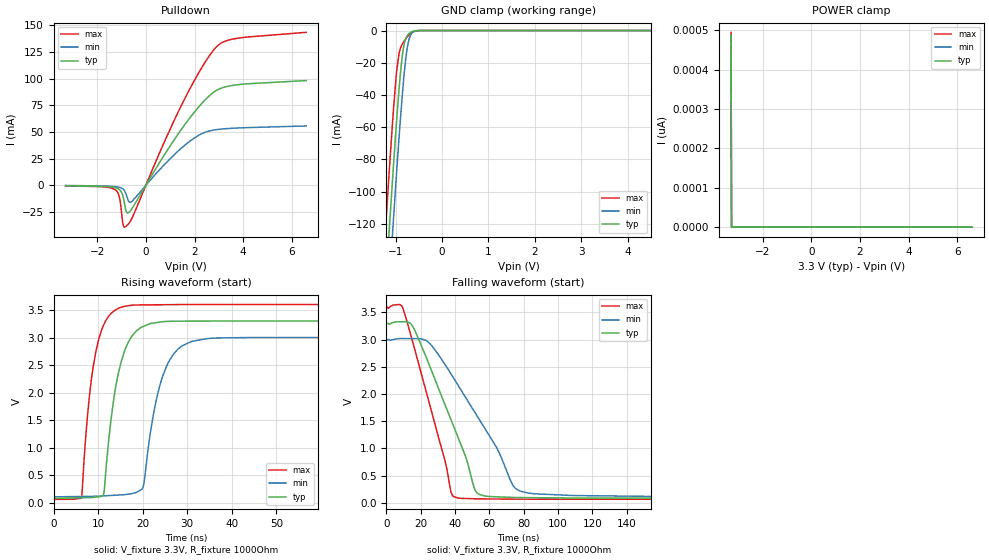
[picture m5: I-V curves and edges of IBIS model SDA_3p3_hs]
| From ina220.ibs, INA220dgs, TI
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|   Model
[Model]   SDA_3p3_hs
Model_type   I/O_open_drain
Polarity   Non-Inverting
Enable   Active-Low
Vinl = 0.99
Vinh = 2.31
Vmeas = 1.65
Vref = 3.3
Cref = 1pF
Rref = 1000
|   typ   min   max
C_comp   2.2433820E-12   1.9359850E-12 2.5433970E-12
[Voltage Range]   3.3   3   3.6
[Temperature Range]   27   85   -40
[Pullup Reference]   3.3   3   3.6
[Pulldown Reference]   -0   -0   -0
[Power Clamp Reference]   3.3   3   3.6
[GND Clamp Reference]   -0   -0   -0
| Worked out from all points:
|   slope of the pulldown table from 0 to 0.495 V, typ, clamps not added: 26.3 ohm
|   GND clamp passes 1 mA (typ) near -0.67 V on its own axis
|   falling waveform, V_fixture 3.3V, R_fixture 1000Ohm: 20-80 % time 24ns typ, 32.2ns min, 18.3ns max; typ from 3.3 V to 0.083 V
|   rising waveform, V_fixture 3.3V, R_fixture 1000Ohm: 20-80 % time 3.66ns typ, 4.29ns min, 3.08ns max; typ from 0.083 V to 3.3 V
[Pulldown]
|   Voltage   I(typ)   I(min)   I(max)
-3.3V     -316.9uA   -207.5uA   -421.7uA
-1.261V   -2.207mA   -1.204mA   -4.07mA
-1.102V   -3.787mA   -1.819mA   -9.812mA
-973.5mV  -7.834mA   -2.97mA    -31.07mA
-914.1mV  -12.66mA   -4.043mA   -38.45mA
-825mV    -23.31mA   -7.395mA   -38.56mA
-696.3mV  -25.37mA   -15.33mA   -35.64mA
-587.4mV  -22.38mA   -15.34mA   -31.61mA
1.393V    50.19mA    33.45mA    71.66mA
2.848V    88.14mA    51.94mA    128.4mA
3.61V     93.68mA    53.5mA     137.1mA
6.59V     98.07mA    55.57mA    143.2mA
[GND Clamp]
|   Voltage   I(typ)   I(min)   I(max)
-3.3V     -1.176A    -1.208A    -1.142A
-1.221V   -162.6mA   -196.9mA   -125.6mA
-1.132V   -122mA     -156mA     -85.52mA
-1.073V   -95.72mA   -129.4mA   -60.19mA
-1.053V   -87.15mA   -120.6mA   -52.17mA
-973.5mV  -54.4mA    -86.43mA   -24.47mA
-924mV    -35.97mA   -66.11mA   -14.02mA
-854.7mV  -15.61mA   -39.98mA   -8.368mA
-805.2mV  -7.274mA   -24.13mA   -6.138mA
-755.7mV  -3.503mA   -12.19mA   -4.229mA
-646.8mV  -706.8uA   -1.595mA   -1.161mA
6.59V     0A         0A         0A
[POWER Clamp]
|   Voltage   I(typ)   I(min)   I(max)
-3.3V     487.8pA    443.7pA    495.1pA
-3.28V    0A         0A         0A
-3.27V    0A         0A         0A
6.59V     0A         0A         0A
[Ramp]
R_load = 1000
|   typ   min   max
dV/dt_r   1.93018/3.63163e-09   1.73473/4.27769e-09   2.12159/3.05717e-09
dV/dt_f   1.93018/2.39503e-08   1.73472/3.22284e-08   2.12159/1.82753e-08
[Falling Waveform]
V_fixture = 3.3V
V_fixture_min = 3V
V_fixture_max = 3.6V
R_fixture = 1000Ohm
C_fixture = 0F
|   Time   V(typ)   V(min)   V(max)
0s        3.3V       3V         3.6V
9.87ns    3.328V     3.02V      3.56V
15.51ns   3.236V     3.018V     2.943V
24.31ns   2.59V      2.959V     1.919V
37.73ns   1.525V     2.368V     193.6mV
41.2ns    1.249V     2.191V     92.2mV
52.96ns   177.5mV    1.593V     73.04mV
73.53ns   98.79mV    332.4mV    68.26mV
82.9ns    95.13mV    179mV      66.67mV
500ns     83.03mV    108.8mV    64.01mV
[Rising Waveform]
V_fixture = 3.3V
V_fixture_min = 3V
V_fixture_max = 3.6V
R_fixture = 1000Ohm
C_fixture = 0F
|   Time   V(typ)   V(min)   V(max)
0s        83.03mV    108.8mV    64.01mV
6.271ns   93.22mV    115.7mV    84.71mV
8.552ns   96.93mV    118.2mV    2.277V
11.18ns   138.1mV    126mV      3.217V
14ns      2.127V     139.5mV    3.505V
17.62ns   3.028V     169mV      3.588V
20.06ns   3.2V       278.2mV    3.592V
25.57ns   3.293V     2.514V     3.597V
34.56ns   3.299V     2.982V     3.6V
500ns     3.3V       3V         3.6V
